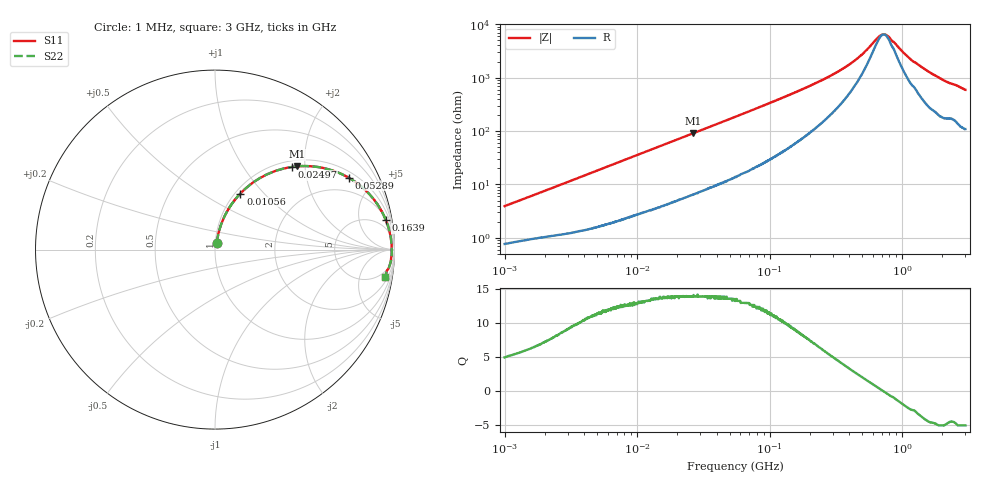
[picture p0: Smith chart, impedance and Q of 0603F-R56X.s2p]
!s-Parameter Generated by FASTRON Sdn. Bhd.
!FASTRON P/N : 0603F-R56X
!Keysight Technologies: E4991B_MY54100416_A.01.15
!Date: Thu Jun 20 13:32:46 2024
!Version  :Rev00  Thu Jun 20 13:32:46 2024
!Data & Calibration Information:
!Freq  S11  S21  S12  S22
!PortZ  Port1:50+j0  Port2:50+j0
!When reading reference impedance value at option line is always used.
! Remarks : This data is being provided solely for informational purposes.
# Hz S dB R 50
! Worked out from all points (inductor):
!   1601 points, 1 MHz to 3 GHz, reference 50 ohm
!   read as one part in series: L = 608 nH near 1.041 MHz
!   highest Q = 14 at 26.51 MHz (marker M1), where L = 545 nH
!   self-resonance near 726 MHz
!   S11 on the Smith chart (normalised r, x): 1 MHz: 1.02, +0.08; 10.56 MHz: 1.06, +0.75; 24.97 MHz: 1.12, +1.71; 52.89 MHz: 1.26, +3.55; 163.9 MHz: 2, +11; 3 GHz: 3, -12
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1000000  -28.20 76.5  -0.07 -2.2  -0.07 -2.2  -28.20 76.5
3804036  -17.30 76.6  -0.20 -7.8  -0.20 -7.8  -17.30 76.6
6696013  -12.70 72.0  -0.41 -13.3  -0.41 -13.3  -12.70 72.0
1.05579e7  -9.30 65.6  -0.78 -20.0  -0.78 -20.0  -9.30 65.6
1.447069e7  -7.13 59.8  -1.25 -26.0  -1.25 -26.0  -7.13 59.8
2.49671e7  -4.02 47.0  -2.69 -38.9  -2.69 -38.9  -4.02 47.0
2.651225e7  -3.74 45.5  -2.92 -40.4  -2.92 -40.4  -3.74 45.5
3.707242e7  -2.42 36.9  -4.41 -49.0  -4.41 -49.0  -2.42 36.9
5.288691e7  -1.46 28.3  -6.46 -57.5  -6.46 -57.5  -1.46 28.3
5.504702e7  -1.38 27.4  -6.71 -58.3  -6.71 -58.3  -1.38 27.4
9.079332e7  -0.66 17.7  -10.30 -67.5  -10.30 -67.5  -0.66 17.7
1.63867e8  -0.30 9.9  -15.30 -73.6  -15.30 -73.6  -0.30 9.9
2.083556e8  -0.24 7.6  -17.50 -74.6  -17.50 -74.6  -0.24 7.6
3.140564e8  -0.17 4.5  -21.90 -73.6  -21.90 -73.6  -0.17 4.5
4.114912e8  -0.15 2.9  -25.50 -69.7  -25.50 -69.7  -0.15 2.9
5.102796e8  -0.14 1.7  -29.30 -61.2  -29.30 -61.2  -0.14 1.7
6.855309e8  -0.13 0.3  -35.90 -17.5  -35.90 -17.5  -0.13 0.3
7.38967e8  -0.13 -0.1  -36.30 5.5  -36.30 5.5  -0.13 -0.1
7.925923e8  -0.13 -0.4  -35.40 26.0  -35.40 26.0  -0.13 -0.4
1.212752e9  -0.16 -2.6  -26.20 67.4  -26.20 67.4  -0.16 -2.6
2.000286e9  -0.23 -5.9  -19.60 72.9  -19.60 72.9  -0.23 -5.9
3e9  -0.38 -9.2  -15.80 70.2  -15.80 70.2  -0.38 -9.2
